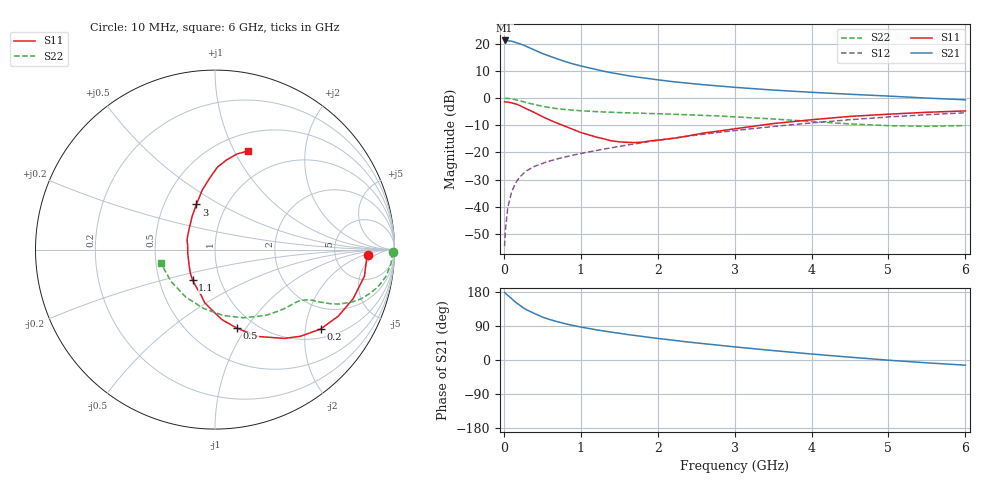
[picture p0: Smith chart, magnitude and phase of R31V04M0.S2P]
! SIEMENS Small Signal Semiconductors
! BFR181
! Si NPN RF Bipolar Junction Transistor in SOT23
! VCE = 1 V  IC = 4 mA
! Common Emitter S-Parameters:  May  1996
# GHz  S  MA  R  50
!  f  S11  S21  S12  S22
! GHz  MAG  ANG  MAG  ANG  MAG  ANG  MAG  ANG
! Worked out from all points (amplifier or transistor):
!   36 points, 10 MHz to 6 GHz, reference 50 ohm
!   highest |S21| = 21.1 dB at 10 MHz (marker M1)
!   |S21| within 3 dB of that: start of sweep to 357.8 MHz
!   unconditionally stable (mu >= 1): 1.097 GHz to 3.255 GHz
!   at 250 MHz: K = 0.38, MSG = 23.7 dB, |S12| = -27.8 dB
!   at 1.4 GHz: K = 1.07, MAG = 12.1 dB, |S12| = -18.3 dB
!   at 6 GHz: K = 0.89, MSG = 2.4 dB, |S12| = -5.4 dB
!   S11 on the Smith chart (normalised r, x): 10 MHz: 12, -3; 200 MHz: 1.26, -2.43; 500 MHz: 0.83, -0.91; 1.1 GHz: 0.74, -0.27; 3 GHz: 0.72, +0.39; 6 GHz: 0.69, +1.14
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0.01  0.8542 -2.1  11.41 178.3  0.0019 85.4  0.9907 -0.9
0.02  0.8459 -4.1  11.35 176.1  0.0037 80.7  0.9872 -1.9
0.05  0.8457 -10.1  11.27 170.9  0.0095 85.0  0.9838 -4.6
0.1  0.8168 -19.6  11.06 162.1  0.0187 79.0  0.9645 -8.9
0.15  0.7804 -28.4  10.51 152.9  0.0271 74.2  0.9306 -13.0
0.2  0.7365 -36.9  9.988 145.6  0.0345 71.4  0.8953 -15.9
0.25  0.6782 -45.4  9.428 138.1  0.0406 67.5  0.8581 -18.7
0.3  0.6271 -52.1  8.772 132.0  0.0464 65.4  0.8196 -20.8
0.4  0.5399 -63.7  7.605 122.5  0.0557 61.6  0.7586 -23.6
0.5  0.4559 -74.2  6.581 113.5  0.0628 59.9  0.707 -25.2
0.6  0.3928 -84.2  5.844 106.5  0.0699 59.2  0.6662 -26.2
0.8  0.3016 -101.0  4.661 95.6  0.0829 58.7  0.6141 -27.4
0.9  0.2651 -107.0  4.226 91.1  0.0894 58.9  0.5981 -28.0
1.1  0.2117 -125.9  3.598 83.4  0.1021 59.5  0.5722 -29.4
1.3  0.1782 -142.3  3.103 76.5  0.1154 60.1  0.5537 -30.8
1.6  0.1535 -172.4  2.594 67.4  0.1367 60.4  0.5354 -33.6
2.2  0.1813 143.6  1.994 52.2  0.1827 59.3  0.5034 -41.3
3  0.272 112.4  1.573 34.6  0.2523 55.0  0.4508 -55.0
3.5  0.3392 102.1  1.4 24.9  0.2998 51.0  0.4123 -67.1
4.5  0.4597 88.3  1.172 7.4  0.3998 40.4  0.3341 -100.9
5.5  0.547 77.0  0.997 -7.5  0.4941 27.4  0.3026 -144.4
6  0.5798 71.4  0.927 -13.7  0.5355 20.3  0.3117 -166.6
